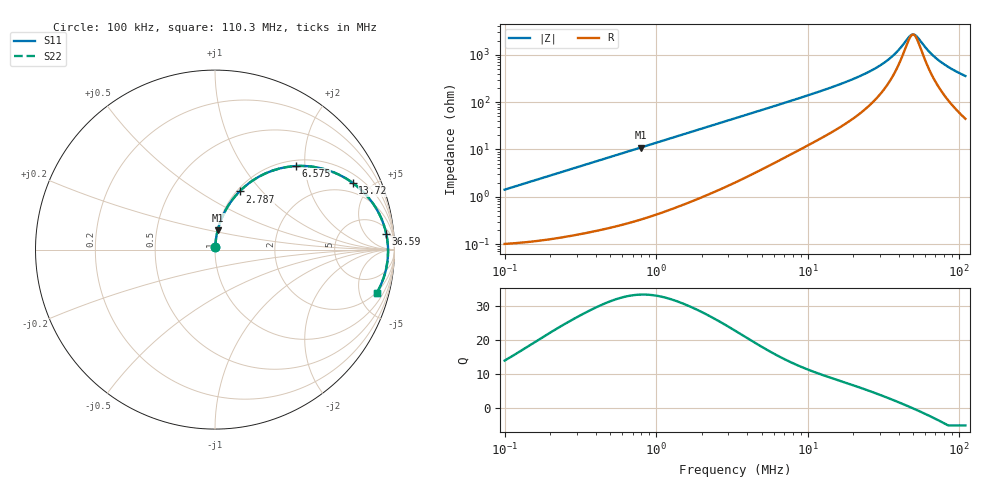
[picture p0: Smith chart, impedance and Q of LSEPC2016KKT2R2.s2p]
! LSEPC2016KKT2R2  S-PARAMETER MODEL  ( General Type )
! Model Generated by TAIYO YUDEN Corporation (http://www.ty-top.com)
! Version 1.0
! TAIYO YUDEN Control No. 180907NI43SB-FBB
! Copyright(c) 2018 TAIYO YUDEN CO.,LTD. All Rights Reserved.
! Product Description (link to TY-COMPAS)
! https://ds.yuden.co.jp/TYCOMPAS/or/detail?pn=LSEPC2016KKT2R2M&u=M
! Products Name : Inductors
! Characteristics :
!  Inductance : 2.2 uH , SRF(min) : -Hz , DC Resistance(max) : 0.1 Ohm
!  Rated Current : Saturation :2300 mA , Temp Rise : 2300 mA (40 degC)
!  Case Size : 2.0 x 1.6 / 0.079 x 0.063 [mm/inch] , Thickness : 1 / 0.039 [mm/inch]
!  (Conditions: Temperature = 25 degC , DC Bias Current/Voltage = 0A / 0V)
! External Node Assignments :
!  1  o---GGG---o  2
! GND o---------o GND
! Frequency Range : 0.1MHz  -  110.285862MHz  [ 402 STEP ]
# MHz S RI R 50
! Freq[MHz].  S11 Real  S11 Imag  S21 Real  S21 Imag  S12 Real  S12 Imag  S22 Real  S22 Imag
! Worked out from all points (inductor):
!   401 points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, 100 kHz to 110.3 MHz, reference 50 ohm
!   read as one part in series: L = 2.25 uH near 103.6 kHz
!   highest Q = 33.3 at 789.8 kHz (marker M1), where L = 2.21 uH
!   self-resonance near 49.74 MHz
!   S11 on the Smith chart (normalised r, x): 100 kHz: 1.00, +0.03; 2.787 MHz: 1.03, +0.76; 6.575 MHz: 1.12, +1.79; 13.72 MHz: 1.42, +3.87; 36.59 MHz: 8, +18; 110.3 MHz: 1.89, -7.08
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0.1  0.00121 0.0141  0.9988 -0.0141  0.9988 -0.0141  0.00121 0.0141
0.323312  0.00368 0.045  0.9963 -0.045  0.9963 -0.045  0.00368 0.045
0.789848  0.015 0.1075  0.985 -0.1075  0.985 -0.1075  0.015 0.1075
1.045308  0.0246 0.1403  0.9754 -0.1403  0.9754 -0.1403  0.0246 0.1403
1.799034  0.0646 0.2293  0.9354 -0.2293  0.9354 -0.2293  0.0646 0.2293
2.787385  0.1369 0.3241  0.8631 -0.3241  0.8631 -0.3241  0.1369 0.3241
3.320932  0.1815 0.3641  0.8185 -0.3641  0.8185 -0.3641  0.1815 0.3641
4.882008  0.317 0.4387  0.683 -0.4387  0.683 -0.4387  0.317 0.4387
6.575149  0.4503 0.4654  0.5497 -0.4654  0.5497 -0.4654  0.4503 0.4654
10.73698  0.6744 0.4249  0.3256 -0.4249  0.3256 -0.4249  0.6744 0.4249
13.72051  0.7673 0.3716  0.2327 -0.3716  0.2327 -0.3716  0.7673 0.3716
23.61378  0.9041 0.2191  0.0959 -0.2191  0.0959 -0.2191  0.9041 0.2191
29.13675  0.9337 0.1567  0.0663 -0.1567  0.0663 -0.1567  0.9337 0.1567
34.71395  0.9501 0.105  0.0499 -0.105  0.0499 -0.105  0.9501 0.105
36.58668  0.9538 0.0896  0.0462 -0.0896  0.0462 -0.0896  0.9538 0.0896
46.75318  0.9635 0.0181  0.0365 -0.0181  0.0365 -0.0181  0.9635 0.0181
50.14601  0.9642 -0.00238  0.0358 0.00238  0.0358 0.00238  0.9642 -0.00238
52.85125  0.9641 -0.0177  0.0359 0.0177  0.0359 0.0177  0.9641 -0.0177
62.96776  0.9601 -0.0694  0.0399 0.0694  0.0399 0.0694  0.9601 -0.0694
73.71824  0.9513 -0.1167  0.0487 0.1167  0.0487 0.1167  0.9513 -0.1167
89.3808  0.9328 -0.176  0.0672 0.176  0.0672 0.176  0.9328 -0.176
110.2859  0.9011 -0.2422  0.0989 0.2422  0.0989 0.2422  0.9011 -0.2422
